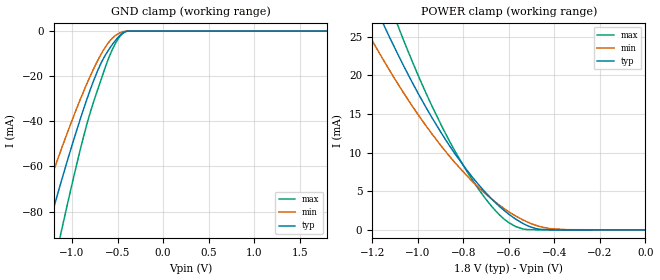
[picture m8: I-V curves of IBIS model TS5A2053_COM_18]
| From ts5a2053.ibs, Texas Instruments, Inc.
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[Model]   TS5A2053_COM_18
Model_type  Terminator
| variable   typ   min   max
C_comp   12.47pF   11.04pF   14.07pF
| C_tri-state   12.47pF   11.04pF   14.07pF
[Temperature Range]   40   100   -40
| Ambient temperature   25   85   -40
[Voltage range]   1.8   1.65   1.95
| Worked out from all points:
|   GND clamp passes 1 mA (typ) near -0.45 V on its own axis
|   POWER clamp passes 1 mA (typ) near -0.55 V on its own axis
[GND Clamp]
| TS5A2053_COM_18
|   Voltage   I(typ)   I(min)   I(max)
-5.5V     -821.7mA   -663.9mA   -1.071A
-1.455V   -115.9mA   -91.97mA   -153.2mA
-1.405V   -108.3mA   -85.87mA   -143.4mA
-1.26V    -86.83mA   -68.58mA   -115.3mA
-1.125V   -67.59mA   -53.14mA   -90.12mA
-1.08V    -61.37mA   -48.16mA   -81.96mA
-880mV    -35.35mA   -27.42mA   -47.82mA
-765mV    -22.18mA   -16.9mA    -31.59mA
-675mV    -13.7mA    -9.809mA   -20.77mA
-565mV    -6.351mA   -3.466mA   -8.846mA
-430mV    -571.7uA   -181.6uA   -636.3uA
1.8V      493.1pA    149.7nA    4.141nA
[POWER Clamp]
| TS5A2053_COM_18
|   Voltage   I(typ)   I(min)   I(max)
-5.5V     607mA      489.7mA    781.5mA
-1.225V   31.53mA    25.85mA    37.74mA
-1.155V   26.92mA    22.22mA    31.82mA
-1.125V   25.04mA    20.73mA    29.4mA
-1.09V    22.91mA    19.05mA    26.67mA
-965mV    15.94mA    13.54mA    17.81mA
-835mV    9.807mA    8.668mA    10.13mA
-730mV    5.77mA     5.425mA    5.166mA
-620mV    2.515mA    2.757mA    1.393mA
-540mV    873.4uA    1.333mA    144.9uA
-460mV    73.42uA    411.3uA    16.81uA
-95.1fV   493.1pA    4.024nA    11.34nA
